PROGRAM PRG_AdvanceHome
VAR
	bEnable									:BOOL;
	bLimitSitchHomeCMD						:BOOL;
	bBusy									:BOOL;
	bDone									:BOOL;
	bError									:BOOL;
	bInput2									:BOOL;
	bInput3									:BOOL;
	bReset									:BOOL;
	bStatusHomed							:BOOL;
	bErrorID								:UDINT;
	iLimitSitchHomeStep						:INT;
	LimitSwitchSignal						:MC_Ref_Signal_Ref;
	mcHomingParameter						:MC_HomingParameter;
	mcStepLimitSwitch						: MC_StepLimitSwitch;
	mcFinishHoming							: MC_FinishHoming;
	mcPower									: MC_Power;
	mcReset									: MC_Reset;
	fbRTrig									:R_TRIG;
	bLimitSwitchBusy						:BOOL;
	bLimitSwitchDone						:BOOL;
	bFinishHomingBusy						:BOOL;
	bFinishHomingDone						:BOOL;
	iTimeout								:INT;
	bHomeCMD								:BOOL;
	mcHome									: MC_Home;
	mcStepAbsoluteSwitch					: MC_StepAbsoluteSwitch;	
	mcStop									: MC_Stop;
	mcAbortHoming							: MC_AbortHoming;
	mcStepBlock: MC_StepBlock;
END_VAR
//StepAbsoluteSwitch
VAR
	bAdvancedHomeAbnormal					:BOOL;
	bStepAbsoluteSwitchCMD					:BOOL;
	iStepAbsoluteSwitchStep					:INT;
	//StepAbsoluteSwitchPara					:
	fbRtrigAbsoluteSwitch					:R_TRIG;
	StepAbsoluteSwitch_Ref_Signal			:MC_Ref_Signal_Ref;
	
	//monitor
	bStepAbsoluteSwitchBusy					:BOOL;
	bStepAbsoluteSwitchDone					:BOOL;
	rAdvancedDonePos						:LREAL;//获取---StepAbsoluteSwitch回完原点坐标，然后在Finsh再返回，确保当前位置是0位
	bHomed									:BOOL;
	
END_VAR
//StepBlock

VAR
	bStepBlockCMD							:BOOL;
	bStepBlockBusy							:BOOL;
	bStepBlockDone							:BOOL;
	iStepBlockStep							:INT;
	rDriverTorque							:LREAL;
	fbRTrigStepBlock						:R_TRIG;
END_VAR

///////Edit BY Gavin 
//////2023-05-29
/////BECKHOFF XI'AN

bInput2													:=iDigitalInput.2;//原点信号
bInput3													:=iDigitalInput.3;//正向限位信号

LimitSwitchSignal.Level									:=bInput3;				//正向限位信号指向限位回原点功能块
mcStepLimitSwitch.Options.DisableDriveAccess			:=FALSE;					//第三方驱动器需置真
mcFinishHoming.Options.DisableDriveAccess				:=FALSE;					//第三方驱动器需置真
bEnable													:=TRUE;					
bStatusHomed											:=Axis_X.NcToPlc.StateDWord.1;//回零状态
mcPower(
			Axis:=Axis_X , 
			Enable:=bEnable,
			Override:= 100,  );
IF bBusy THEN
	mcPower( 
			Axis:=Axis_X ,
			Enable_Positive:=TRUE , 
			Enable_Negative:= TRUE, );
ELSE
	mcPower(
			Axis:=Axis_X ,  
			Enable_Positive:=NOT bInput3 ,
			Enable_Negative:= TRUE,  );
END_IF
		
		
//////////////////////////////////////////////////////////////////////	
//限位回原点	
A_LimitSwitchHome();

bLimitSwitchBusy				:=mcStepLimitSwitch.Busy;
bLimitSwitchDone				:=mcStepLimitSwitch.Done;
bFinishHomingBusy				:=mcFinishHoming.Busy;
bFinishHomingDone				:=mcFinishHoming.Done;

///////////////////////////////////////////////////////////////////////////
//原点加限位回原点
mcStepAbsoluteSwitch.Options.DisableDriveAccess				:=FALSE;
StepAbsoluteSwitch_Ref_Signal.Level							:=bInput2;
A_StepAbsoluteSwitchHome();

bStepAbsoluteSwitchBusy					:=mcStepAbsoluteSwitch.Busy;
bStepAbsoluteSwitchDone					:=mcStepAbsoluteSwitch.Done;
////////////////////////////////////////////////////////////////////////////
//撞死回原点
A_StepBlockHome();
bStepBlockBusy							:=mcStepBlock.Busy;
bStepBlockDone							:=mcStepBlock.Done;
rDriverTorque							:=Axis_X.NcToPlc.ActTorque;
//////////////////////////////////////////////////////////////////////////
mcFinishHoming(
	Axis:=Axis_X , 
	Parameter:=mcHomingParameter ,
	Distance:=0-rAdvancedDonePos ,    
	Velocity:=10 , 
	Acceleration:= , 
	Deceleration:= , 
	Jerk:= , 
	BufferMode:= , 
	Options:= , 
	Done=> , 
	Busy=> , 
	CommandAborted=> , 
	Error=> , 
	ErrorID=> );
	
Axis_X.ReadStatus();	
bHomed				:=Axis_X.Status.Homed;


mcStop(Axis:=Axis_X , Execute:= );

mcAbortHoming(
	Axis:=Axis_X , 
	Parameter:=mcHomingParameter , 
	Options:= , 
	Done=> , 
	Busy=> , 
	CommandAborted=> , 
	Error=> , 
	ErrorID=> );

ACTION A_LimitSwitchHome:
fbRTrig(CLK:=bLimitSitchHomeCMD);
//必须定义到CASE外面，在case里面，有问题。不执行。
mcStepLimitSwitch(
	Axis:=Axis_X , 
	Parameter:=mcHomingParameter , 
	Direction:=mcPositiveDirection , 
	LimitSwitchMode:=mcRisingEdge , 
	LimitSwitchSignal:=LimitSwitchSignal , 
	Velocity:=10 , 
	Acceleration:= , 
	Deceleration:= , 
	Jerk:= , 
	SetPosition:=0 , 
	TimeLimit:=T#1000S , 
	DistanceLimit:=100000000 , 
	TorqueLimit:=100 , 
	BufferMode:= , 
	Options:= , 
	Done=> , 
	Busy=> , 
	Active=> , 
	CommandAborted=> , 
	Error=> , 
	ErrorID=> );






CASE iLimitSitchHomeStep OF
	0:
		IF fbRTrig.Q THEN
			iLimitSitchHomeStep				:=iLimitSitchHomeStep+1;
		END_IF
	1:
		bBusy							:=TRUE;
		bError							:=FALSE;
		bDone							:=FALSE;
		mcStepLimitSwitch(Axis:=Axis_X , Parameter:=mcHomingParameter , Execute:=FALSE);
		mcFinishHoming(Axis:=Axis_X , Parameter:=mcHomingParameter , Execute:=FALSE  );
		mcAbortHoming(Axis:=Axis_X , Parameter:=mcHomingParameter , Execute:=FALSE);
		iLimitSitchHomeStep				:=10;
	10://因为 mcStepLimitSwitch.Done信号很短，如果在CASE里面用，Execute信号等mcStepLimitSwitch.Done完成再置Flase
		mcStepLimitSwitch(Axis:=Axis_X ,Parameter:=mcHomingParameter , Execute:=TRUE);
		IF mcStepLimitSwitch.Busy THEN
			iLimitSitchHomeStep				:=iLimitSitchHomeStep+1;
		END_IF
	11:
		IF NOT mcStepLimitSwitch.Busy THEN
			IF  mcStepLimitSwitch.Error OR   mcStepLimitSwitch.CommandAborted  THEN
				iLimitSitchHomeStep				:=990;
			ELSE
				IF  mcStepLimitSwitch.Done THEN
					iLimitSitchHomeStep				:=iLimitSitchHomeStep+1;
				END_IF
			END_IF
		END_IF
	12:
		rAdvancedDonePos				:=Axis_X.NcToPlc.ActPos;
		mcStepLimitSwitch(Axis:=Axis_X ,Parameter:=mcHomingParameter , Execute:=FALSE);
		iLimitSitchHomeStep				:=iLimitSitchHomeStep+1;
	13:
		mcFinishHoming(Axis:=Axis_X , Parameter:=mcHomingParameter , Execute:=TRUE);
		IF mcFinishHoming.Busy THEN
			iLimitSitchHomeStep				:=iLimitSitchHomeStep+1;
		END_IF
	14:
		
		IF NOT mcFinishHoming.Busy THEN
			IF mcFinishHoming.Error OR mcFinishHoming.CommandAborted THEN
				iLimitSitchHomeStep				:=990;
			ELSE
				IF mcFinishHoming.Done THEN
					iLimitSitchHomeStep				:=iLimitSitchHomeStep+1;
				END_IF
			END_IF
		END_IF
	15:
		mcFinishHoming(Axis:=Axis_X , Parameter:=mcHomingParameter , Execute:=FALSE);
		iLimitSitchHomeStep				:=20;
	20:
		bBusy							:=FALSE;
		bDone							:=TRUE;
		IF NOT bLimitSitchHomeCMD THEN
			iLimitSitchHomeStep				:=0;
		END_IF
	990:
		mcAbortHoming(Axis:=Axis_X , Parameter:=mcHomingParameter , Execute:=TRUE);
		IF mcAbortHoming.Busy THEN
			iLimitSitchHomeStep				:=iLimitSitchHomeStep+1;
		END_IF
	991:
		mcAbortHoming(Axis:=Axis_X , Parameter:=mcHomingParameter , Execute:=FALSE);
		IF NOT mcAbortHoming.Busy THEN
			iLimitSitchHomeStep				:=iLimitSitchHomeStep+1;
		END_IF
	992:
		iLimitSitchHomeStep					:=999;
	999:
		bBusy							:=FALSE;
		bDone							:=FALSE;
		bError							:=TRUE;
		mcStepLimitSwitch(Axis:=Axis_X , Parameter:=mcHomingParameter , Execute:=FALSE);
		mcFinishHoming(Axis:=Axis_X , Parameter:=mcHomingParameter , Execute:=FALSE  );
		iLimitSitchHomeStep				:=0;
END_CASE
END_ACTION

ACTION A_StepAbsoluteSwitchHome:
mcStepAbsoluteSwitch(
	Axis:=Axis_X , 
	Parameter:=mcHomingParameter , 
	Direction:=mcPositiveDirection , 
	SwitchMode:=mcRisingEdge , 
	ReferenceSignal:=StepAbsoluteSwitch_Ref_Signal , 
	Velocity:=10 , 
	Acceleration:= , 
	Deceleration:= , 
	Jerk:= , 
	SetPosition:=0 , 
	TimeLimit:=T#1000S , 
	DistanceLimit:=1000000 , 
	TorqueLimit:=100 , 
	PositiveLimitSwitch:=bInput3 , 
	NegativeLimitSwitch:= , 
	BufferMode:= , 
	Options:= , 
	Done=> , 
	Busy=> , 
	Active=> , 
	CommandAborted=> , 
	Error=> , 
	ErrorID=> );	

fbRtrigAbsoluteSwitch(CLK:=bStepAbsoluteSwitchCMD);
CASE iStepAbsoluteSwitchStep OF
	0:
		IF fbRtrigAbsoluteSwitch.Q THEN
			iStepAbsoluteSwitchStep						:=iStepAbsoluteSwitchStep+1;
		END_IF
	1://初始化
		bBusy									:=TRUE;
		bAdvancedHomeAbnormal					:=FALSE;
		bError									:=FALSE;
		bDone									:=FALSE;
		iTimeout								:=0;
		mcStepAbsoluteSwitch(Axis:=Axis_X , Parameter:=mcHomingParameter , Execute:=FALSE);
		mcFinishHoming(Axis:=Axis_X , Parameter:=mcHomingParameter , Execute:=FALSE  );
		mcAbortHoming(Axis:=Axis_X , Parameter:=mcHomingParameter , Execute:=FALSE);
		iStepAbsoluteSwitchStep					:=10;
	10://mcStepAbsoluteSwitch
		mcStepAbsoluteSwitch(Axis:=Axis_X , Parameter:=mcHomingParameter , Execute:=TRUE);
		IF mcStepAbsoluteSwitch.Busy THEN
			iStepAbsoluteSwitchStep						:=iStepAbsoluteSwitchStep+1;
		END_IF
	11:
		IF NOT mcStepAbsoluteSwitch.Busy THEN
			IF mcStepAbsoluteSwitch.Error OR mcStepAbsoluteSwitch.CommandAborted THEN
				iStepAbsoluteSwitchStep						:=990;
			ELSE
				IF mcStepAbsoluteSwitch.Done THEN
					iStepAbsoluteSwitchStep						:=iStepAbsoluteSwitchStep+1;
				END_IF
			END_IF
			iTimeout									:=0;
		ELSE
			IF iTimeout>10000 THEN
				iTimeout								:=0;
				iStepAbsoluteSwitchStep					:=990;
			ELSE
				iTimeout								:=iTimeout+1;
			END_IF
		END_IF
	12://因为DONE信号很短，故Done信号完成，再将Execute置False。如果EXE一直为真，那么Done也一直为真、
		rAdvancedDonePos							:=Axis_X.NcToPlc.ActPos;
		mcStepAbsoluteSwitch(Axis:=Axis_X , Parameter:=mcHomingParameter , Execute:=FALSE);
		iStepAbsoluteSwitchStep						:=20;
	20://mcFinishHoming
		mcFinishHoming(Axis:=Axis_X , Parameter:=mcHomingParameter , Execute:=TRUE  );
		IF mcFinishHoming.Busy THEN
			iStepAbsoluteSwitchStep						:=iStepAbsoluteSwitchStep+1;
		END_IF
	21:
		IF NOT mcFinishHoming.Busy THEN
			IF mcFinishHoming.Error OR mcFinishHoming.CommandAborted THEN
				iStepAbsoluteSwitchStep						:=990;
			ELSE
				IF mcFinishHoming.Done THEN
					iStepAbsoluteSwitchStep						:=iStepAbsoluteSwitchStep+1;
				END_IF
			END_IF
			iTimeout									:=0;
		ELSE
			IF iTimeout>10000 THEN
				iTimeout								:=0;
				iStepAbsoluteSwitchStep					:=990;
			ELSE
				iTimeout								:=iTimeout+1;
			END_IF
		END_IF
	22:
		mcFinishHoming(Axis:=Axis_X , Parameter:=mcHomingParameter , Execute:=FALSE  );
		iStepAbsoluteSwitchStep						:=30;
	30:
		bBusy										:=FALSE;
		bDone										:=TRUE;
		IF NOT bStepAbsoluteSwitchCMD THEN
			iStepAbsoluteSwitchStep						:=0;
		END_IF
	990://异常中断时，高级回原点应用终止
		bAdvancedHomeAbnormal						:=TRUE;
		iStepAbsoluteSwitchStep						:=997;
	997:
		mcAbortHoming(Axis:=Axis_X , Parameter:=mcHomingParameter , Execute:=TRUE);
		IF mcAbortHoming.Busy THEN
			iStepAbsoluteSwitchStep						:=iStepAbsoluteSwitchStep+1;
		END_IF
	998:
		mcAbortHoming(Axis:=Axis_X , Parameter:=mcHomingParameter , Execute:=FALSE);
		IF NOT mcAbortHoming.Busy THEN
			iStepAbsoluteSwitchStep						:=iStepAbsoluteSwitchStep+1;
		END_IF
	999://异常处理
		bBusy										:=FALSE;
		bDone										:=FALSE;
		bError										:=TRUE;
		iTimeout									:=0;
		mcStepAbsoluteSwitch(Axis:=Axis_X , Parameter:=mcHomingParameter , Execute:=FALSE);
		mcFinishHoming(Axis:=Axis_X , Parameter:=mcHomingParameter , Execute:=FALSE  );
		mcAbortHoming(Axis:=Axis_X , Parameter:=mcHomingParameter , Execute:=FALSE);
		iStepAbsoluteSwitchStep						:=0;
END_CASE
END_ACTION

ACTION A_StepBlockHome:
mcStepBlock(
	Axis:=Axis_X , 
	Parameter:=mcHomingParameter ,  
	Direction:=mcPositiveDirection , 
	Velocity:=10 , 
	Acceleration:= , 
	Deceleration:= , 
	Jerk:= , 
	SetPosition:=0 , 
	DetectionVelocityLimit:=10 , 
	DetectionVelocityTime:=T#2S , 
	TimeLimit:=T#100S , 
	DistanceLimit:=100000 , 
	TorqueLimit:=30 , 
	TorqueTolerance:=5 , 
	BufferMode:= , 
	Options:= , 
	Done=> , 
	Busy=> , 
	Active=> , 
	CommandAborted=> , 
	Error=> , 
	ErrorID=> );

fbRTrigStepBlock(CLK:=bStepBlockCMD);	
CASE iStepBlockStep OF
	0:
		IF fbRTrigStepBlock.Q THEN
			iStepBlockStep						:=iStepBlockStep+1;
		END_IF
	1:
		bBusy									:=TRUE;
		bAdvancedHomeAbnormal					:=FALSE;
		bError									:=FALSE;
		bDone									:=FALSE;
		iTimeout								:=0;
		mcStepBlock(Axis:=Axis_X , Parameter:=mcHomingParameter , Execute:=FALSE);
		mcFinishHoming(Axis:=Axis_X , Parameter:=mcHomingParameter , Execute:=FALSE  );
		mcAbortHoming(Axis:=Axis_X , Parameter:=mcHomingParameter , Execute:=FALSE);
		iStepBlockStep						:=10;
	10:
		mcStepBlock(Axis:=Axis_X , Parameter:=mcHomingParameter , Execute:=TRUE);
		IF mcStepBlock.Busy THEN
			iStepBlockStep						:=iStepBlockStep+1;
		END_IF
	11:
		IF NOT mcStepBlock.Busy THEN
			IF mcStepBlock.Error OR mcStepBlock.CommandAborted THEN
				iStepBlockStep						:=990;
			ELSE
				IF mcStepBlock.Done THEN
					iStepBlockStep					:=iStepBlockStep+1;
				END_IF
			END_IF
			iTimeout								:=0;
		ELSE
			IF iTimeout>10000 THEN
				iTimeout							:=0;
				iStepAbsoluteSwitchStep				:=990;
			ELSE
				iTimeout							:=iTimeout+1;
			END_IF
		END_IF
	12:
		mcStepBlock(Axis:=Axis_X , Parameter:=mcHomingParameter , Execute:=FALSE);
		iStepBlockStep					:=20;
	20:
		mcFinishHoming(Axis:=Axis_X , Parameter:=mcHomingParameter , Execute:=TRUE  );
		IF mcFinishHoming.Busy THEN
			iStepBlockStep						:=iStepBlockStep+1;
		END_IF
	21:
		IF NOT mcFinishHoming.Busy THEN
			IF mcFinishHoming.Error OR mcFinishHoming.CommandAborted THEN
				iStepBlockStep						:=990;
			ELSE
				IF mcFinishHoming.Done THEN
					iStepBlockStep						:=iStepBlockStep+1;
				END_IF
			END_IF
		ELSE
			IF iTimeout>10000 THEN
				iTimeout							:=0;
				iStepAbsoluteSwitchStep				:=990;
			ELSE
				iTimeout							:=iTimeout+1;
			END_IF
		END_IF
	22:
		mcFinishHoming(Axis:=Axis_X , Parameter:=mcHomingParameter , Execute:=FALSE  );
		iStepBlockStep						:=30;
	30:
		bBusy								:=FALSE;
		bDone								:=TRUE;
		IF NOT bStepBlockCMD THEN
			iStepBlockStep					:=0;
		END_IF
	990:
		mcAbortHoming(Axis:=Axis_X , Parameter:=mcHomingParameter , Execute:=TRUE);
		IF mcAbortHoming.Busy THEN
			iStepBlockStep					:=iStepBlockStep+1;
		END_IF
	991:
		mcAbortHoming(Axis:=Axis_X , Parameter:=mcHomingParameter , Execute:=FALSE);
		IF NOT mcAbortHoming.Busy THEN
			iStepBlockStep					:=iStepBlockStep+1;
		END_IF
	992:
		iStepBlockStep						:=999;
	999:
		bBusy								:=FALSE;
		bDone								:=FALSE;
		bError								:=TRUE;
		mcStepBlock(Axis:=Axis_X , Parameter:=mcHomingParameter , Execute:=FALSE);
		mcFinishHoming(Axis:=Axis_X , Parameter:=mcHomingParameter , Execute:=FALSE  );
		iStepBlockStep						:=0;
END_CASE
END_ACTION

END_PROGRAM
